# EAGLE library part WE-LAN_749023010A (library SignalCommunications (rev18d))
LAN-Transformer WE-LAN 10/10/1000 Base Tx - Compliant with IEEE 802.3 standards - SMD -- Ethernet -- Power over Ethernet -- 1 Gigabit Ethernet -- Compliant with most IC's for ethernet applications like Intel, AMD, Globespan and Realtek -- Hub, Router, Switch Details see: http://katalog.we-online.de/en/pbs/WE-LAN/S/749023010A? Updated by Dan Xu 2014-07-08 2014 (C) Würth Elektronik
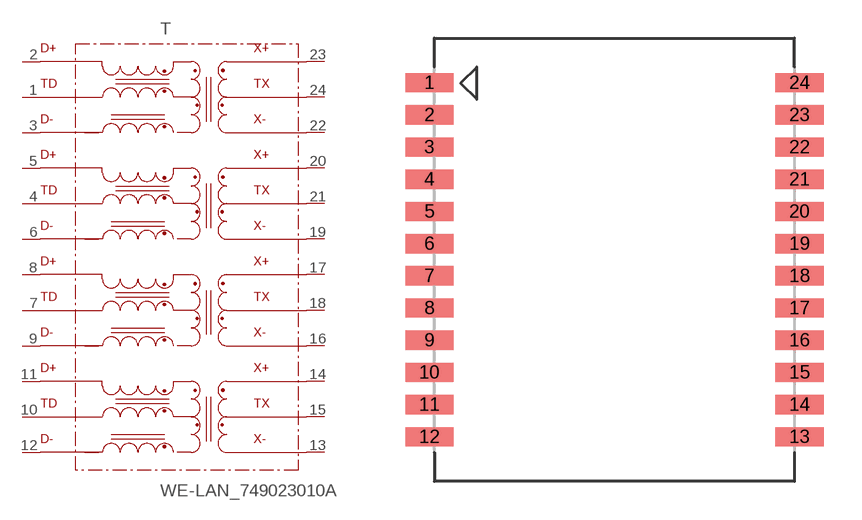
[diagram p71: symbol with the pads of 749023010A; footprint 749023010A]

Designator prefix T

## WE-LAN_749023010A  [749023010A]
1  1
2  2
3  3
4  4
5  5
6  6
7  7
8  8
9  9
10  10
11  11
12  12
13  13
14  14
15  15
16  16
17  17
18  18
19  19
20  20
21  21
22  22
23  23
24  24

## Footprint 749023010A (pad centres in mm)
MAX Height = 6.5 mm
smd 1.9 x 0.76: 1 -7.3,6.985; 2 -7.3,5.715; 3 -7.3,4.445; 4 -7.3,3.175; 5 -7.3,1.905; 6 -7.3,0.635; 7 -7.3,-0.635; 8 -7.3,-1.905; 9 -7.3,-3.175; 10 -7.3,-4.445; 11 -7.3,-5.715; 12 -7.3,-6.985; 13 7.3,-6.985; 14 7.3,-5.715; 15 7.3,-4.445; 16 7.3,-3.175; 17 7.3,-1.905; 18 7.3,-0.635; 19 7.3,0.635; 20 7.3,1.905; 21 7.3,3.175; 22 7.3,4.445; 23 7.3,5.715; 24 7.3,6.985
